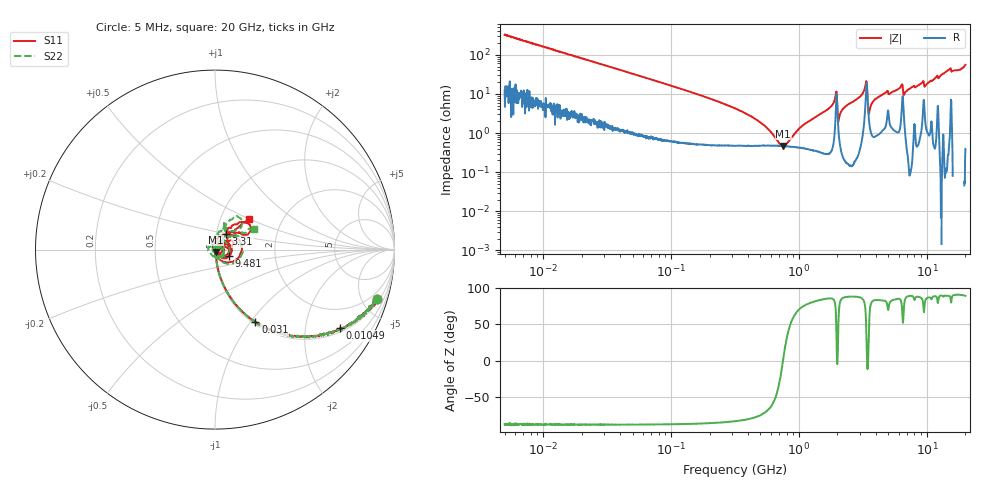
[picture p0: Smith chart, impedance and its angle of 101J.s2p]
!Keysight Technologies,P5008B,MY61100088,A.16.20.02
!Date: Wednesday, November 08, 2023 15:25:00
!Correction: S11(C  2-Port  )
!S21(C  2-Port  )
!S12(C  2-Port  )
!S22(C  2-Port  )
!S2P File: Measurements: S11, S21, S12, S22:Log Frequency Sweep
# Hz S  dB  R 50
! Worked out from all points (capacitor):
!   1601 points, 5 MHz to 20 GHz, reference 50 ohm
!   read as one part in series: C = 98.5 pF near 5.212 MHz
!   lowest |Z| = 464 mohm at 751.6 MHz (marker M1)
!   series resonance near 749.9 MHz, so ESL is about 460 pH
!   S11 on the Smith chart (normalised r, x): 5 MHz: 1.24, -6.48; 10.49 MHz: 1.15, -3.09; 31 MHz: 1.03, -1.06; 3.31 GHz: 1.11, +0.19; 9.481 GHz: 1.17, -0.09; 20 GHz: 1.36, +0.49
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5000000  -0.48 -16.9  -10.71 70.9  -10.71 70.9  -0.48 -16.9
1.049311e7  -1.71 -32.1  -5.49 55.0  -5.50 55.0  -1.71 -32.1
1.995555e7  -4.08 -49.8  -2.34 38.7  -2.34 38.7  -4.08 -49.8
3.100439e7  -6.73 -60.7  -1.18 27.4  -1.18 27.4  -6.73 -60.8
7.964482e7  -13.95 -76.7  -0.23 11.4  -0.24 11.4  -13.97 -76.7
3.162278e8  -26.37 -81.6  -0.05 2.2  -0.05 2.2  -26.67 -82.8
7.515623e8  -37.08 -72.2  -0.05 -0.7  -0.05 -0.7  -39.59 -74.5
9.638885e8  -41.58 -61.8  -0.05 -1.5  -0.05 -1.5  -48.19 -69.7
1.120248e9  -46.02 -47.0  -0.05 -2.1  -0.05 -2.1  -69.47 13.3
1.2621e9  -49.22 -37.6  -0.05 -2.5  -0.06 -2.5  -55.28 113.1
1.414562e9  -53.01 54.9  -0.05 -3.0  -0.06 -3.0  -45.53 94.8
1.930631e9  -25.78 65.4  -0.26 -6.7  -0.26 -6.7  -25.76 59.6
2.197766e9  -48.42 146.0  -0.07 -4.6  -0.08 -4.6  -47.77 148.6
3.31004e9  -19.56 54.1  -0.59 -12.0  -0.59 -12.0  -19.55 46.7
3.866979e9  -52.64 119.6  -0.10 -7.8  -0.10 -7.8  -40.70 -8.7
5.037181e9  -31.91 14.9  -0.22 -10.4  -0.22 -10.4  -30.31 1.2
6.46025e9  -20.41 -4.1  -0.81 -14.5  -0.82 -14.4  -25.62 -11.0
8.458946e9  -40.89 9.7  -0.09 -18.7  -0.09 -18.7  -41.86 164.6
9.480792e9  -21.12 -25.1  -0.59 -20.4  -0.60 -20.4  -24.92 -46.3
1.04621e10  -27.80 -18.1  -0.06 -23.5  -0.06 -23.5  -34.89 143.7
1.450274e10  -14.19 43.4  -0.11 -35.3  -0.12 -35.3  -14.43 61.4
2e10  -11.97 41.8  -0.37 -55.1  -0.37 -55.1  -12.20 27.2
